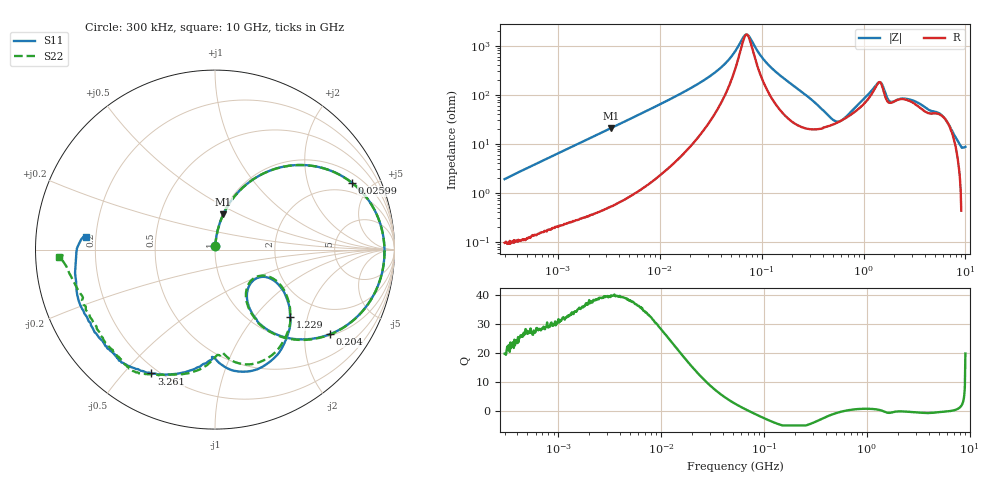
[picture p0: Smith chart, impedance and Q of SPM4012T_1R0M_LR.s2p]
! S-Parameter Data Generated by TDK Corporation
! Copyright(C) 2019 TDK Corporation.
! All Rights Reserved.
! TDK P/N: SPM4012T-1R0M-LR (Inductor)
! Property: L=1uH at 100kHz
! Size(LxWxT): 4.4x4.1x1.2mm
! Model Type: s2p (Touchstone File Format Version 1.0)
! Frequency: DC=Yes Start=0.3MHz Stop=10000MHz 802points Log-sweep
! Model Generated on Sep. 23, 2019
! Port Assignments:
!  1 ---@@@--- 2
! Applicable Conditions:
!  Temperature = 25 degC
!  DC Bias Current = 0 A
!  Small Signal Operation
! Terms and conditions regarding TDK Simulation Models
! (1)This simulation model is being provided solely for informational purposes. Please refer to the specifications of the products in terms of detailed characteristics of such products.
! (2)In no event shall TDK Corporation of any of its subsidiaries be liable for any loss or damage arising, directly or indirectly,
!  From any information contained in this simulation model, including, but not limited to loss or damages arising from any inaccuracies, omissions or errors in connection with such information.
! (3)Any and all copyrights on this simulation model are owned by TDK Corporation.
!  Duplication or redistribution of this simulation model without prior written permission from TDK Corporation is prohibited.
! (4)This simulation model is subject to any modification or change without any prior notice.
! (5)Neither TDK Corporation nor any of its subsidiaries shall make any warranty, express or implied,
!  Including but not limited to the correctness, implied warranties of merchantability and fitness for a particular purpose with respect to this simulation models.
! (6)The use of this simulation model shall be deemed to have consented to the terms and conditions hereof.
# Hz S MA R 50
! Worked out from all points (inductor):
!   801 points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, 300 kHz to 10 GHz, reference 50 ohm
!   read as one part in series: L = 1.02 uH near 318.3 kHz
!   highest Q = 39.9 at 3.33 MHz (marker M1), where L = 1 uH
!   self-resonance near 71.3 MHz
!   S11 on the Smith chart (normalised r, x): 300 kHz: 1.00, +0.04; 25.99 MHz: 1.43, +3.82; 204 MHz: 1.05, -2.67; 1.229 GHz: 1.42, -1.57; 3.261 GHz: 0.17, -0.60; 10 GHz: 0.16, +0.05
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300000  0.01815 86.1  0.9988 -1.2  0.999 -1.1  0.01783 85.5
1713600  0.1067 82.2  0.9913 -6.2  0.9914 -6.2  0.1067 82.2
3330145  0.2029 76.7  0.9741 -11.8  0.9741 -11.8  0.2029 76.7
9671944  0.5137 56.8  0.8403 -31.2  0.8403 -31.2  0.5136 56.8
1.603896e7  0.7052 41.6  0.6732 -45.4  0.6733 -45.4  0.7052 41.6
2.599165e7  0.8489 26.0  0.4563 -58.7  0.4564 -58.7  0.8489 26.0
4.138262e7  0.9227 12.1  0.2407 -66.2  0.2407 -66.2  0.9228 12.0
5.477226e7  0.9407 4.3  0.1238 -60.3  0.1238 -60.3  0.9407 4.3
7.244865e7  0.9442 -3.1  0.0562 3.8  0.05623 3.8  0.9442 -3.2
1.145169e8  0.9185 -16.2  0.2148 57.5  0.2148 57.5  0.9184 -16.3
2.039737e8  0.7942 -36.5  0.4891 43.7  0.4891 43.7  0.7937 -36.8
3.126428e8  0.6011 -53.0  0.6759 23.9  0.676 23.9  0.5997 -53.4
4.627802e8  0.3769 -59.5  0.7606 1.8  0.7607 1.8  0.3732 -60.0
6.490631e8  0.2728 -41.6  0.7396 -18.6  0.7398 -18.6  0.265 -41.6
9.216398e8  0.3783 -27.9  0.6158 -40.2  0.6159 -40.2  0.3726 -26.7
1.228555e9  0.5632 -42.0  0.4143 -55.0  0.4144 -55.0  0.5575 -41.1
1.459486e9  0.6886 -61.4  0.283 -41.1  0.283 -41.1  0.6681 -61.6
1.767019e9  0.6377 -87.3  0.4215 -34.6  0.4215 -34.7  0.5928 -84.3
3.261479e9  0.776 -117.2  0.2883 -61.3  0.2882 -61.3  0.7773 -116.2
6.172341e9  0.8111 -142.9  0.2488 -89.4  0.2491 -89.6  0.7898 -144.1
7.875699e9  0.7941 -167.0  0.2159 -110.9  0.2162 -111.0  0.8033 -166.0
1e10  0.7206 174.2  0.1602 -124.9  0.1603 -125.1  0.8683 -177.3
